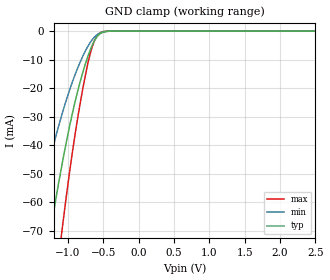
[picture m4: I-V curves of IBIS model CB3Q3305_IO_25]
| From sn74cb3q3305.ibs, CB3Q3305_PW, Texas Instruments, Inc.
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[Model]   CB3Q3305_IO_25
Model_type  Terminator
| variable   typ   min   max
C_comp   3.55pF   2.97pF   3.83pF
| C_tri-state   3.55pF   2.97pF   3.83pF
[Temperature Range]   40   100   -40
| Ambient temperature   25   85   -40
[Voltage range]   2.5   2.3   2.7
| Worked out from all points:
|   GND clamp passes 1 mA (typ) near -0.55 V on its own axis
[GND Clamp]
| CB3Q3305_IO_25
|   Voltage   I(typ)   I(min)   I(max)
-5.5V     -1.002A    -757.8mA   -1.259A
-1.49V    -110mA     -70.56mA   -161.2mA
-1.255V   -71.31mA   -44.92mA   -106.2mA
-1.23V    -67.51mA   -42.45mA   -100.6mA
-1.095V   -48.22mA   -30.06mA   -72.04mA
-1.075V   -45.57mA   -28.37mA   -68.03mA
-935mV    -28.59mA   -17.66mA   -42.09mA
-775mV    -13.22mA   -8.022mA   -18.2mA
-655mV    -4.871mA   -2.955mA   -5.38mA
-550mV    -1.008mA   -714.3uA   -673.7uA
-350mV    -6.625uA   -9.714uA   -757.7nA
2.5V      147.2pA    716.2pA    14.5pA
